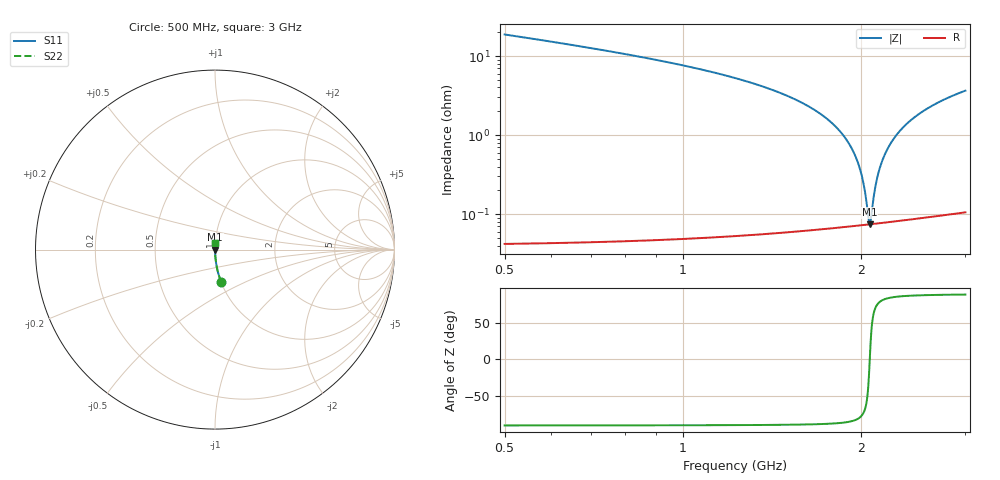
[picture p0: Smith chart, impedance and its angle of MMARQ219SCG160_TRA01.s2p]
! MMARQ219SCG160_TRA01  S-PARAMETER MODEL  ( General Type )
! Model Generated by TAIYO YUDEN Corporation (http://www.ty-top.com)
! Version 1.0
! TAIYO YUDEN Control No. 180601
! Copyright(c) 2018 TAIYO YUDEN CO.,LTD. All Rights Reserved.
! Product Description (link to TY-COMPAS)
! https://ds.yuden.co.jp/TYCOMPAS/or/detail?pn=MMARQ219SCG160JTRA01&u=M
! Products Name : Multilayer Ceramic Capacitors
! Characteristics :
!  Capacitance : 16 pF , Rated Voltage : 250V , TCC : CG / C0G
!  Case Size : 2.0 x 1.25 / 0.079 x 0.049 [mm/inch] , Thickness : 0.85 / 0.033 [mm/inch]
!  (Conditions: Temperature = 25 degC , DC Bias Current/Voltage = 0A / 0V)
! External Node Assignments :
!  1  o---| |---o  2
! GND o---------o GND
! Frequency Range : 500MHz  -  3000MHz  [ 401 STEP ]
# MHz S RI R 50
! Freq[MHz].  S11 Real  S11 Imag  S21 Real  S21 Imag  S12 Real  S12 Imag  S22 Real  S22 Imag
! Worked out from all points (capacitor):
!   401 points, 500 MHz to 3 GHz, reference 50 ohm
!   read as one part in series: C = 16 pF near 512.5 MHz
!   lowest |Z| = 74.3 mohm at 2.069 GHz (marker M1)
!   series resonance near 2.068 GHz, so ESL is about 370 pH
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500  0.0343 -0.1809  0.9657 0.1809  0.9657 0.1809  0.0343 -0.1809
918.75  0.00796 -0.0862  0.992 0.0862  0.992 0.0862  0.00796 -0.0862
1337.5  0.00241 -0.0431  0.9976 0.0431  0.9976 0.0431  0.00241 -0.0431
1575  0.00131 -0.0265  0.9987 0.0265  0.9987 0.0265  0.00131 -0.0265
1750  0.000911 -0.0161  0.9991 0.0161  0.9991 0.0161  0.000911 -0.0161
1868.75  0.000779 -0.00975  0.9992 0.00975  0.9992 0.00975  0.000779 -0.00975
1956.25  0.000737 -0.00534  0.9993 0.00534  0.9993 0.00534  0.000737 -0.00534
1987.5  0.000733 -0.00382  0.9993 0.00382  0.9993 0.00382  0.000733 -0.00382
2012.5  0.000732 -0.00262  0.9993 0.00262  0.9993 0.00262  0.000732 -0.00262
2031.25  0.000734 -0.00173  0.9993 0.00173  0.9993 0.00173  0.000734 -0.00173
2056.25  0.000739 -0.000561  0.9993 0.000561  0.9993 0.000561  0.000739 -0.000561
2068.75  0.000742 2.03e-05  0.9993 -2.03e-05  0.9993 -2.03e-05  0.000742 2.03e-05
2081.25  0.000746 0.000598  0.9993 -0.000598  0.9993 -0.000598  0.000746 0.000598
2106.25  0.000756 0.00174  0.9992 -0.00174  0.9992 -0.00174  0.000756 0.00174
2125  0.000766 0.00259  0.9992 -0.00259  0.9992 -0.00259  0.000766 0.00259
2168.75  0.000793 0.00455  0.9992 -0.00455  0.9992 -0.00455  0.000793 0.00455
2237.5  0.000851 0.00754  0.9991 -0.00754  0.9991 -0.00754  0.000851 0.00754
2325  0.000948 0.0112  0.9991 -0.0112  0.9991 -0.0112  0.000948 0.0112
2443.75  0.00112 0.016  0.9989 -0.016  0.9989 -0.016  0.00112 0.016
2587.5  0.00138 0.0216  0.9986 -0.0216  0.9986 -0.0216  0.00138 0.0216
2775  0.00179 0.0285  0.9982 -0.0285  0.9982 -0.0285  0.00179 0.0285
3000  0.00238 0.0363  0.9976 -0.0363  0.9976 -0.0363  0.00238 0.0363
